PROGRAM p01_FBD
VAR
	S0: BOOL;
	S1: BOOL;
	S2: BOOL;
	S3: BOOL;
	L0: BOOL;
	L1: BOOL;
	L2: BOOL;
	pomnilnaCelica: SR;
END_VAR

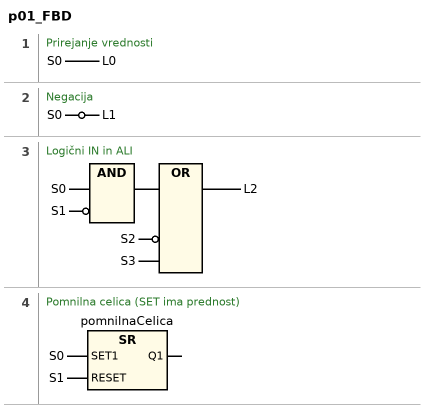
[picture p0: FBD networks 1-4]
// NETWORK 1
// Prirejanje vrednosti
L0 := S0;

// NETWORK 2
// Negacija
L1 := NOT S0;

// NETWORK 3
// Logični IN in ALI
L2 := S0 AND NOT S1 OR NOT S2 OR S3;

// NETWORK 4
// Pomnilna celica (SET ima prednost)
pomnilnaCelica(SET1 := S0, RESET := S1); // SR

END_PROGRAM
